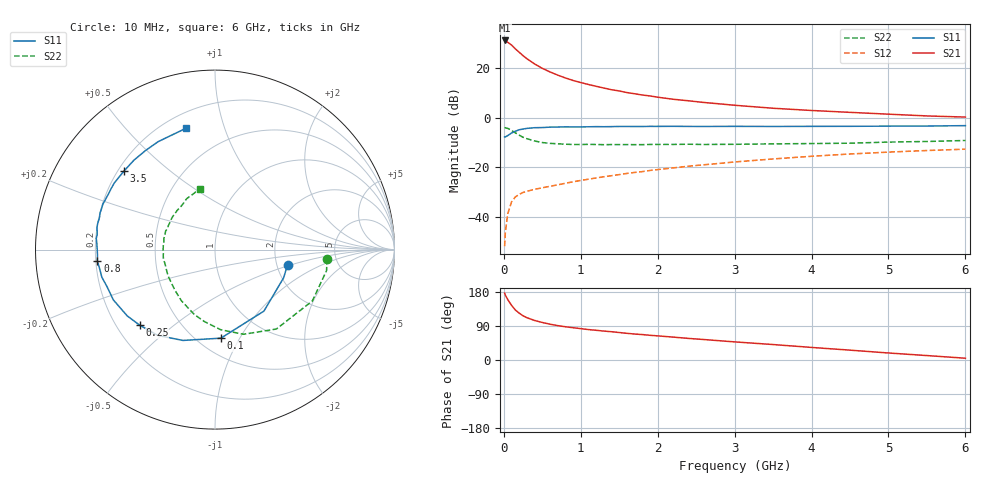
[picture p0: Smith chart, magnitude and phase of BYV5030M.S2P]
! SIEMENS Small Signal Semiconductors
! BFY420
! Si NPN RF SIEGET Grounded Emitter Transistor in MICRO-X
! VCE = 0.5 V  IC = 30 mA
! Common Emitter S-Parameters:  October  1996
# GHz  S  MA  R  50
!  f  S11  S21  S12  S22
! GHz  MAG  ANG  MAG  ANG  MAG  ANG  MAG  ANG
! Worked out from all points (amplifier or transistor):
!   36 points, 10 MHz to 6 GHz, reference 50 ohm
!   highest |S21| = 31.2 dB at 10 MHz (marker M1)
!   |S21| within 3 dB of that: start of sweep to 137.2 MHz
!   unconditionally stable (mu >= 1): start of sweep to 31.7 MHz; 712.3 MHz to end of sweep
!   at 250 MHz: K = 0.56, MSG = 27.5 dB, |S12| = -30.1 dB
!   at 1.4 GHz: K = 1.27, MAG = 14.2 dB, |S12| = -23.3 dB
!   at 6 GHz: K = 1.30, MAG = 3.2 dB, |S12| = -12.6 dB
!   S11 on the Smith chart (normalised r, x): 10 MHz: 2.29, -0.47; 100 MHz: 0.64, -0.84; 250 MHz: 0.29, -0.38; 800 MHz: 0.21, -0.05; 3.5 GHz: 0.22, +0.36; 6 GHz: 0.29, +0.75
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0.01  0.4132 -11.8  36.13 176.3  0.0026 96.7  0.6262 -4.7
0.02  0.4133 -22.4  35.73 171.1  0.005 88.0  0.6325 -10.6
0.05  0.4379 -51.5  33.2 159.8  0.0116 75.4  0.6133 -27.8
0.1  0.4945 -86.2  29.23 144.3  0.0202 61.0  0.5592 -52.3
0.15  0.5366 -109.4  24.43 131.9  0.0255 53.1  0.498 -71.3
0.2  0.5747 -123.7  20.91 123.6  0.0288 47.6  0.4477 -85.9
0.25  0.5944 -134.9  17.81 116.6  0.0314 43.9  0.405 -98.4
0.3  0.6128 -142.9  15.49 111.6  0.0331 43.4  0.3798 -107.6
0.4  0.632 -153.7  12.15 104.3  0.0364 41.6  0.3412 -123.2
0.5  0.6363 -161.2  9.913 99.0  0.0389 42.7  0.3177 -134.8
0.6  0.6489 -166.3  8.394 94.5  0.0418 43.4  0.3055 -142.8
0.7  0.6517 -170.8  7.253 90.7  0.0446 44.9  0.3002 -150.1
0.8  0.6586 -174.5  6.349 87.7  0.048 45.6  0.2941 -156.2
0.9  0.6555 -177.3  5.652 85.2  0.0515 46.5  0.2901 -161.7
1.1  0.6595 176.9  4.686 80.3  0.058 48.3  0.2922 -169.6
1.3  0.6617 172.7  3.977 76.3  0.065 48.7  0.2877 -176.5
1.6  0.6696 167.3  3.223 70.4  0.0759 48.9  0.2889 175.6
2.2  0.6741 158.0  2.366 60.4  0.0981 47.1  0.2911 163.6
3.5  0.6699 139.1  1.558 40.8  0.1484 38.1  0.2986 143.1
4.5  0.6742 125.0  1.288 26.0  0.1868 27.6  0.3081 126.6
5.5  0.6828 109.9  1.091 11.7  0.2195 16.5  0.3337 111.0
6  0.6955 103.3  1.035 4.7  0.2336 11.0  0.3495 104.3
